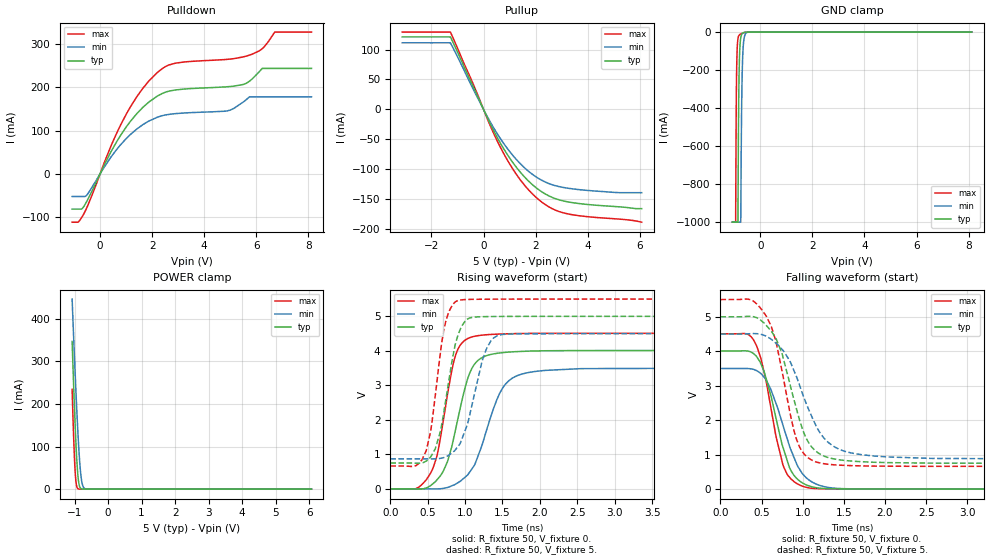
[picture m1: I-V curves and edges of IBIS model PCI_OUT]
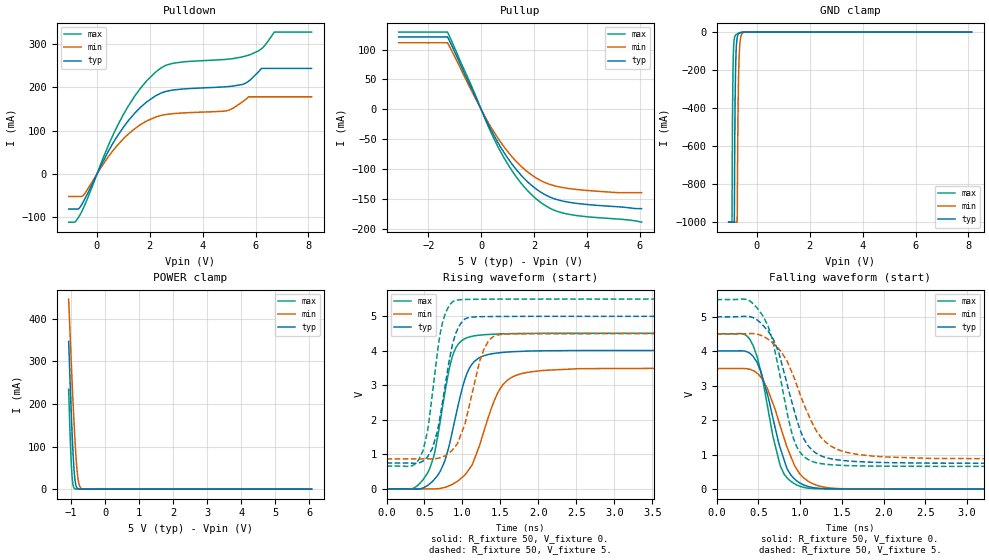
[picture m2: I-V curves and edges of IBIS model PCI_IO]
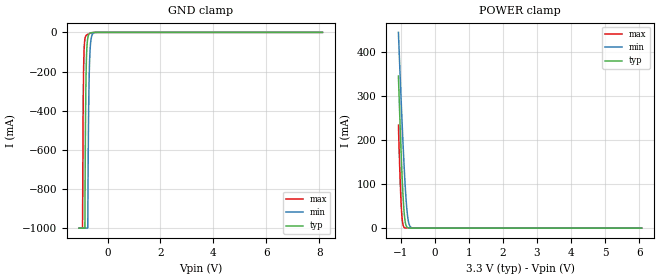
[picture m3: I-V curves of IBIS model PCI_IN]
|   IBIS Model for Tsi382 PBGA Package
[IBIS Ver]   3.2
[Disclaimer] This model is subject to change.
   Integrated Device Technology, Inc. ("IDT") hereby grants the
   user of this IBIS model a non-exclusive, nontransferable
   license to use this IBIS model under the following terms. The
   user is granted this license only to use the IBIS model and is
   not granted rights to sell, copy (except as needed to run the
   IBIS model), rent, lease or sub-license the IBIS model in
   whole or in part, or in modified form to anyone. The User may
   modify the IBIS model to suit its specific applications, but
   rights to derivative works and such modifications shall belong
   to IDT. This IBIS model is provided on an AS IS" basis and IDT
   makes absolutely no warranty with respect to the information
   contained herein. IDT DISCLAIMS AND CUSTOMER WAIVES ALL
   WARRANTIES, EXPRESS AND IMPLIED, INCLUDING WARRANTIES OF
   MERCHANTABILITY AND FITNESS FOR A PARTICULAR PURPOSE. THE
   ENTIRE RISK AS TO QUALITY AND PERFORMANCE IS WITH THE USER
   ACCORDINGLY, IN NO EVENT SHALL IDT BE LIABLE FOR ANY DIRECT OR
   INDIRECT DAMAGES, WHETHER IN CONTRACT OR TORT, INCLUDING ANY
   LOST PROFITS OR OTHER INCIDENTAL, CONSEQUENTIAL, EXEMPLARY, OR
   PUNITIVE DAMAGES ARISING OUT OF THE USE OR APPLICATION OF THE
   IBIS model. Further, IDT reserves the right to make changes
   without notice to any product herein to improve reliability,
   function, or design. IDT does not convey any license under
   patent rights or any other intellectual property rights,
   including those of third parties. IDT is not obligated to
   provide maintenance or support for the licensed IBIS model.
[Copyright]   Copyright 2009, Integrated Device Technology, Inc. all
   rights reserved.
[File Name]   tsi382_5vpci_pbga.ibs
[File Rev]   1.1
[Source]   Developed by:
   Tundra Semiconductor
   603 March Rd.
   Ottawa ON,  K2K 2M5
   www.tundra.com
[Notes]
   Revision History
   Rev 1.0
   - 02/25/2009 Inital Release. IBIS model generated from
   SPICE model extraction. AP
   Rev 1.1
   - 08/31/2009, Updated with IDT formatting. IT
[Component] Tsi382
[Manufacturer] Integrated Device Technology, Inc.
|   typ   min   max
[Package]
R_pkg   218m   168m   293m
L_pkg   3.31nH   2.38nH   5.22nH
C_pkg   0.61pF   0.39pF   1.00pF
[Pin]  signal_name   model_name   R_pin   L_pin   C_pin
E9   GPIO[0]   NC   236.1m   4.0nh   0.67pf
D8   GPIO[1]   NC   212.2m   2.7nh   0.48pf
C9   GPIO[2]   NC   234.6m   3.5nh   0.63pf
D9   GPIO[3]   NC   216.8m   2.8nh   0.52pf
K4   JTAG_TCK   JTAG_IN   260.7m   4.2nh   0.79pf
M3   JTAG_TDI   JTAG_IN   201.1m   2.9nh   0.49pf
K3   JTAG_TDO   JTAG_OUT   199.0m   2.7nh   0.43pf
M12   JTAG_TMS   JTAG_IN   226.1m   3.3nh   0.58pf
K9   JTAG_TRSTn   JTAG_IN   217.8m   3.2nh   0.61pf
B1   PCI_AD[0]   PCI_IO   230.1m   3.2nh   0.65pf
C2   PCI_AD[1]   PCI_IO   218.5m   3.2nh   0.61pf
E1   PCI_AD[10]   PCI_IO   185.3m   2.6nh   0.48pf
G1   PCI_AD[11]   PCI_IO   180.2m   2.5nh   0.45pf
H3   PCI_AD[12]   PCI_IO   221.4m   3.4nh   0.66pf
H1   PCI_AD[13]   PCI_IO   187.1m   2.6nh   0.47pf
H4   PCI_AD[14]   PCI_IO   247.9m   4.2nh   0.80pf
J1   PCI_AD[15]   PCI_IO   197.3m   2.8nh   0.54pf
J5   PCI_AD[16]   PCI_IO   223.4m   3.4nh   0.56pf
J7   PCI_AD[17]   PCI_IO   203.3m   3.1nh   0.63pf
L6   PCI_AD[18]   PCI_IO   199.4m   2.9nh   0.57pf
M6   PCI_AD[19]   PCI_IO   177.7m   2.5nh   0.45pf
F4   PCI_AD[2]   PCI_IO   288.0m   5.2nh   1.00pf
K6   PCI_AD[20]   PCI_IO   217.9m   3.4nh   0.66pf
K7   PCI_AD[21]   PCI_IO   221.0m   3.6nh   0.67pf
M8   PCI_AD[22]   PCI_IO   188.5m   2.8nh   0.50pf
K8   PCI_AD[23]   PCI_IO   231.0m   3.7nh   0.72pf
M10   PCI_AD[24]   PCI_IO   215.9m   3.0nh   0.62pf
L10   PCI_AD[25]   PCI_IO   215.6m   3.1nh   0.65pf
L8   PCI_AD[26]   PCI_IO   168.3m   2.3nh   0.42pf
M11   PCI_AD[27]   PCI_IO   215.8m   3.0nh   0.62pf
H9   PCI_AD[28]   PCI_IO   286.5m   4.9nh   0.98pf
K12   PCI_AD[29]   PCI_IO   202.0m   3.0nh   0.55pf
E3   PCI_AD[3]   PCI_IO   281.6m   4.6nh   0.97pf
J12   PCI_AD[30]   PCI_IO   188.9m   2.7nh   0.50pf
L12   PCI_AD[31]   PCI_IO   222.0m   3.0nh   0.63pf
E2   PCI_AD[4]   PCI_IO   213.7m   3.4nh   0.63pf
F2   PCI_AD[5]   PCI_IO   168.6m   2.4nh   0.43pf
D1   PCI_AD[6]   PCI_IO   200.8m   2.8nh   0.55pf
D3   PCI_AD[7]   PCI_IO   271.0m   4.2nh   0.83pf
F1   PCI_AD[8]   PCI_IO   177.9m   2.5nh   0.44pf
G4   PCI_AD[9]   PCI_IO   236.4m   3.9nh   0.76pf
F3   PCI_CBEn[0]   PCI_IO   222.6m   3.5nh   0.68pf
J3   PCI_CBEn[1]   PCI_IO   243.9m   4.0nh   0.76pf
M4   PCI_CBEn[2]   PCI_IO   190.9m   2.8nh   0.48pf
L9   PCI_CBEn[3]   PCI_IO   227.1m   3.3nh   0.70pf
B12   PCI_CLK   PCI_IN   218.9m   3.1nh   0.59pf
H10   PCI_CLKO[0]   PCI_OUT   246.1m   4.2nh   0.80pf
B2   PCI_CLKO[1]   PCI_OUT   240.6m   3.3nh   0.65pf
J9   PCI_CLKO[2]   PCI_OUT   230.0m   3.2nh   0.57pf
J8   PCI_CLKO[3]   PCI_OUT   276.0m   4.4nh   0.83pf
A12   PCI_CLKO[4]   PCI_OUT   229.3m   3.3nh   0.62pf
M2   PCI_DEVSELn   PCI_IO   225.9m   3.1nh   0.60pf
M5   PCI_FRAMEn   PCI_IO   182.0m   2.6nh   0.46pf
G9   PCI_GNTn[0]   PCI_IO   235.6m   4.0nh   0.76pf
F12   PCI_GNTn[1]   PCI_OUT   178.7m   2.6nh   0.46pf
F11   PCI_GNTn[2]   PCI_OUT   206.3m   3.1nh   0.60pf
E10   PCI_GNTn[3]   PCI_OUT   252.2m   4.1nh   0.82pf
D12   PCI_INTAn   PCI_IN   195.5m   2.7nh   0.54pf
F9   PCI_INTBn   PCI_IN   253.9m   4.4nh   0.84pf
C10   PCI_INTCn   PCI_IN   242.6m   3.9nh   0.75pf
C12   PCI_INTDn   PCI_IN   217.7m   3.2nh   0.59pf
L5   PCI_IRDYn   PCI_IO   205.3m   3.0nh   0.58pf
L3   PCI_LOCKn   PCI_OUT   194.1m   2.7nh   0.48pf
B11   PCI_M66EN   PCI_IN   244.4m   3.5nh   0.71pf
K1   PCI_PAR   PCI_IO   210.2m   2.9nh   0.52pf
J4   PCI_PERRn   PCI_IO   272.8m   4.5nh   0.84pf
H12   PCI_PMEn   PCI_IN   180.5m   2.5nh   0.45pf
F10   PCI_REQn[0]   PCI_IO   204.0m   3.2nh   0.62pf
J10   PCI_REQn[1]   PCI_IN   266.6m   4.2nh   0.82pf
G10   PCI_REQn[2]   PCI_IN   183.1m   2.7nh   0.52pf
H11   PCI_REQn[3]   PCI_IN   204.4m   2.9nh   0.58pf
E12   PCI_RSTn   PCI_OUT   184.7m   2.7nh   0.47pf
J2   PCI_SERRn   PCI_IO   187.1m   2.5nh   0.48pf
J6   PCI_STOPn   PCI_IO   275.1m   5.0nh   0.92pf
K5   PCI_TRDYn   PCI_IO   190.6m   2.7nh   0.53pf
B9   PCIE_PERSTn   NC   254.1m   4.2nh   0.70pf
A8   PCIE_REFCLK_n   NC   188.2m   2.9nh   0.40pf
B8   PCIE_REFCLK_p   NC   188.9m   2.8nh   0.39pf
A11   PCIE_REXT   NC   227.9m   3.5nh   0.75pf
B6   PCIE_RXD_n   NC   190.9m   2.7nh   0.45pf
A6   PCIE_RXD_p   NC   192.5m   2.7nh   0.41pf
B4   PCIE_TXD_n   NC   189.6m   2.9nh   0.41pf
A4   PCIE_TXD_p   NC   186.6m   2.8nh   0.39pf
K11   PWRUP_EN_ARB   GEN33_IN   261.2m   3.8nh   0.82pf
L1   PWRUP_PLL_BYPASS   GEN33_IN   240.0m   3.4nh   0.62pf
A2   SR_CLK   NC   242.9m   3.3nh   0.61pf
D4   SR_CSn   NC   216.3m   2.8nh   0.57pf
A3   SR_DIN   NC   209.3m   2.8nh   0.45pf
E4   SR_DOUT   NC   293.9m   4.8nh   0.88pf
D7   TEST_BCE   NC   225.6m   2.8nh   0.51pf
C3   TEST_BIDR_CTL   NC   216.2m   2.9nh   0.53pf
B3   TEST_ON   NC   223.2m   3.2nh   0.53pf
E5   VDD   POWER
E8   VDD   POWER
F6   VDD   POWER
F7   VDD   POWER
G6   VDD   POWER
G7   VDD   POWER
H5   VDD   POWER
H8   VDD   POWER
D2   VDD_PCI   POWER
D11   VDD_PCI   POWER
E11   VDD_PCI   POWER
G2   VDD_PCI   POWER
G11   VDD_PCI   POWER
H2   VDD_PCI   POWER
J11   VDD_PCI   POWER
K2   VDD_PCI   POWER
L4   VDD_PCI   POWER
L7   VDD_PCI   POWER
L11   VDD_PCI   POWER
B5   VDD_PCIE   POWER
B7   VDD_PCIE   POWER
C4   VDD_PCIE   POWER
C8   VDD_PCIE   POWER
C6   VDDA_PCIE   POWER
D6   VDDA_PCIE   POWER
B10   VDDA_PLL   POWER
C11   VIO_PCI   POWER
L2   VIO_PCI   POWER
M9   VIO_PCI   POWER
A1   VSS   GND
A5   VSS   GND
A7   VSS   GND
A9   VSS   GND
C1   VSS   GND
C5   VSS   GND
C7   VSS   GND
D5   VSS   GND
D10   VSS   GND
E6   VSS   GND
E7   VSS   GND
F5   VSS   GND
F8   VSS   GND
G3   VSS   GND
G5   VSS   GND
G8   VSS   GND
G12   VSS   GND
H6   VSS   GND
H7   VSS   GND
K10   VSS   GND
M1   VSS   GND
M7   VSS   GND
A10   VSSA_PLL   GND
| Models and submodels in the file (6): PCI_OUT (Output), PCI_IO (I/O), PCI_IN (Input), JTAG_IN (Input), JTAG_OUT (Output), GEN33_IN (Input)
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[Model]   PCI_OUT
Model_type  Output
C_comp 4.536p 4.202p 4.874p
Polarity   Non-Inverting
Enable   Active-High
Vmeas =   1.32V
Cref =   10pF
Rref =   50
Vref=   0.0V
[Temperature Range]   27.0   125.0   -40.0
[Voltage Range] 5. 4.5 5.5
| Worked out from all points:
|   slope of the pulldown table from 0 to 0.75 V, typ, clamps not added: 8.81 ohm
|   slope of the pullup table from 0 to 0.75 V, typ, clamps not added: 11.8 ohm
|   GND clamp passes 1 mA (typ) near -0.58 V on its own axis
|   POWER clamp passes 1 mA (typ) near -0.80 V on its own axis
|   rising waveform, R_fixture 50, V_fixture 0.: 20-80 % time 271ps typ, 341ps min, 223ps max; typ from 0 V to 4.01 V
|   rising waveform, R_fixture 50, V_fixture 5.: 20-80 % time 204ps typ, 254ps min, 174ps max; typ from 0.748 V to 5 V
|   falling waveform, R_fixture 50, V_fixture 0.: 20-80 % time 260ps typ, 305ps min, 229ps max; typ from 4.01 V to 0 V
|   falling waveform, R_fixture 50, V_fixture 5.: 20-80 % time 307ps typ, 393ps min, 259ps max; typ from 5 V to 0.748 V
[Pulldown]
-1.072V   -80.93mA   -51.78mA   -111mA
-830.1mV  -80.93mA   -51.78mA   -110.2mA
-625.6mV  -75.05mA   -51.78mA   -92.1mA
425mV     51.67mA    39.35mA    65.16mA
1.011V    108.6mA    81.72mA    138.1mA
2.21V     179.7mA    130.8mA    234.1mA
2.879V    193.3mA    138.9mA    254.9mA
4.887V    200.8mA    145.2mA    263.9mA
5.761V    214.7mA    177.7mA    274.1mA
6.226V    243mA      177.7mA    288.2mA
6.71V     243mA      177.7mA    326.7mA
8.123V    243mA      177.7mA    326.7mA
[Pullup]
-3.123V   121mA      111.2mA    129.1mA
-1.273V   121mA      111.2mA    129.1mA
-408.1mV  39.21mA    34.71mA    43.33mA
103.2mV   -9.96mA    -8.61mA    -11.21mA
754mV     -64.09mA   -55.48mA   -71.94mA
1.433V    -105.7mA   -91.4mA    -118.6mA
1.786V    -121.9mA   -105.2mA   -136.8mA
2.186V    -135.9mA   -116.9mA   -152.8mA
2.725V    -148.2mA   -126.7mA   -167.3mA
3.264V    -154.4mA   -131.5mA   -174.5mA
4.984V    -161.7mA   -138.3mA   -182.2mA
6.072V    -165.4mA   -138.8mA   -188mA
[GND Clamp]
-1.072V   -1A        -1A        -1A
-946.2mV  -1A        -1A        -1A
-927.6mV  -1A        -1A        -477.7mA
-913.6mV  -1A        -1A        -259.6mA
-857.8mV  -1A        -1A        -35.04mA
-829.9mV  -387.1mA   -1A        -20.17mA
-792.7mV  -109.1mA   -1A        -13.52mA
-750.8mV  -31.16mA   -1A        -10.02mA
-718.2mV  -13.49mA   -425.6mA   -7.927mA
-681mV    -5.936mA   -150.7mA   -5.835mA
-541.4mV  -487.9uA   -4.567mA   -875.4uA
8.123V    0A         0A         0A
[Power Clamp]
-1.072V   346.3mA    445.7mA    234.2mA
-1.025V   239mA      352.7mA    117.5mA
-985.9mV  158.9mA    279.6mA    47.19mA
-953.7mV  100.9mA    221.8mA    15.32mA
-930mV    65.56mA    181.6mA    5.554mA
-906.4mV  38.32mA    144mA      1.868mA
-865.6mV  11.54mA    86.96mA    261.8uA
-839.8mV  4.741mA    57.78mA    114.1uA
-809.7mV  1.564mA    32.24mA    114.1uA
-764.6mV  288.3uA    10.74mA    114.1uA
-708.7mV  34.28uA    2.193mA    114.1uA
6.072V    0A         0A         0A
[Ramp]
dV/dt_r 2.406/269.779p 2.1/340.819p 2.705/222.777p
dV/dt_f 2.551/306.834p 2.179/393.351p 2.904/258.7p
[Rising Waveform]
R_fixture = 50
V_fixture = 0.
0s        0V         0V         0V
340ps     -4.676mV   86.06uV    4.549mV
540ps     94.69mV    -2.304mV   456.9mV
640ps     301mV      -2.262mV   1.113V
770ps     822.3mV    41.22mV    2.797V
860ps     1.592V     120.4mV    3.781V
1.06ns    3.349V     481.1mV    4.379V
1.46ns    3.937V     2.758V     4.487V
1.71ns    3.979V     3.291V     4.5V
4.91ns    4.01V      3.5V       4.508V
[Rising Waveform]
R_fixture = 50
V_fixture = 5.
V_fixture_min = 4.5
V_fixture_max = 5.5
0s        748.2mV    868.5mV    660.9mV
340ps     743.4mV    868.5mV    668.5mV
480ps     805.4mV    867.5mV    1.103V
610ps     1.216V     870.6mV    2.858V
720ps     2.281V     911.3mV    4.647V
890ps     4.347V     1.186V     5.445V
1.03ns    4.918V     1.86V      5.488V
1.28ns    4.991V     4.027V     5.496V
1.43ns    4.995V     4.436V     5.498V
4.91ns    5V         4.5V       5.5V
[Falling Waveform]
R_fixture = 50
V_fixture = 0.
0s        4.01V      3.5V       4.508V
400ps     3.94V      3.477V     4.342V
530ps     3.418V     3.25V      3.403V
670ps     2.118V     2.522V     1.6V
760ps     1.216V     1.855V     703.3mV
860ps     527.8mV    1.121V     291.2mV
990ps     192.2mV    470.5mV    92.32mV
1.17ns    40.8mV     141mV      16.71mV
1.44ns    9.292mV    19.45mV    6.614mV
4.91ns    8.688uV    23.08uV    4.321uV
[Falling Waveform]
R_fixture = 50
V_fixture = 5.
V_fixture_min = 4.5
V_fixture_max = 5.5
0s        5V         4.5V       5.5V
370ps     5.012V     4.511V     5.491V
560ps     4.742V     4.432V     5.006V
670ps     4.387V     4.245V     4.331V
740ps     3.99V      4.079V     3.529V
920ps     2.368V     3.287V     1.483V
1.14ns    1.146V     1.95V      809.5mV
1.37ns    882.2mV    1.249V     708.4mV
1.71ns    797.4mV    1.002V     675.1mV
4.91ns    748.3mV    869.1mV    660.9mV
[Model]   PCI_IO
Model_type  I/O
C_comp 4.536p 4.202p 4.874p
Polarity   Non-Inverting
Enable   Active-High
Vinl =   0.80V
Vinh =   2.00V
Vmeas =   1.32V
Cref =   10pF
Rref =   150
Vref=   0.0V
[Temperature Range]   27.0   125.0   -40.0
[Voltage Range] 5. 4.5 5.5
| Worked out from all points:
|   slope of the pulldown table from 0 to 0.75 V, typ, clamps not added: 8.81 ohm
|   slope of the pullup table from 0 to 0.75 V, typ, clamps not added: 11.8 ohm
|   GND clamp passes 1 mA (typ) near -0.58 V on its own axis
|   POWER clamp passes 1 mA (typ) near -0.80 V on its own axis
|   rising waveform, R_fixture 50, V_fixture 0.: 20-80 % time 271ps typ, 341ps min, 223ps max; typ from 0 V to 4.01 V
|   rising waveform, R_fixture 50, V_fixture 5.: 20-80 % time 204ps typ, 254ps min, 174ps max; typ from 0.748 V to 5 V
|   falling waveform, R_fixture 50, V_fixture 0.: 20-80 % time 260ps typ, 305ps min, 229ps max; typ from 4.01 V to 0 V
|   falling waveform, R_fixture 50, V_fixture 5.: 20-80 % time 307ps typ, 393ps min, 259ps max; typ from 5 V to 0.748 V
[Pulldown]
-1.072V   -80.93mA   -51.78mA   -111mA
-830.1mV  -80.93mA   -51.78mA   -110.2mA
-625.6mV  -75.05mA   -51.78mA   -92.1mA
425mV     51.67mA    39.35mA    65.16mA
1.011V    108.6mA    81.72mA    138.1mA
2.21V     179.7mA    130.8mA    234.1mA
2.879V    193.3mA    138.9mA    254.9mA
4.887V    200.8mA    145.2mA    263.9mA
5.761V    214.7mA    177.7mA    274.1mA
6.226V    243mA      177.7mA    288.2mA
6.71V     243mA      177.7mA    326.7mA
8.123V    243mA      177.7mA    326.7mA
[Pullup]
-3.123V   121mA      111.2mA    129.1mA
-1.273V   121mA      111.2mA    129.1mA
-408.1mV  39.21mA    34.71mA    43.33mA
103.2mV   -9.96mA    -8.61mA    -11.21mA
754mV     -64.09mA   -55.48mA   -71.94mA
1.433V    -105.7mA   -91.4mA    -118.6mA
1.786V    -121.9mA   -105.2mA   -136.8mA
2.186V    -135.9mA   -116.9mA   -152.8mA
2.725V    -148.2mA   -126.7mA   -167.3mA
3.264V    -154.4mA   -131.5mA   -174.5mA
4.984V    -161.7mA   -138.3mA   -182.2mA
6.072V    -165.4mA   -138.8mA   -188mA
[GND Clamp]
-1.072V   -1A        -1A        -1A
-946.2mV  -1A        -1A        -1A
-927.6mV  -1A        -1A        -477.7mA
-913.6mV  -1A        -1A        -259.6mA
-857.8mV  -1A        -1A        -35.04mA
-829.9mV  -387.1mA   -1A        -20.17mA
-792.7mV  -109.1mA   -1A        -13.52mA
-750.8mV  -31.16mA   -1A        -10.02mA
-718.2mV  -13.49mA   -425.6mA   -7.927mA
-681mV    -5.936mA   -150.7mA   -5.835mA
-541.4mV  -487.9uA   -4.567mA   -875.4uA
8.123V    0A         0A         0A
[Power Clamp]
-1.072V   346.3mA    445.7mA    234.2mA
-1.025V   239mA      352.7mA    117.5mA
-985.9mV  158.9mA    279.6mA    47.19mA
-953.7mV  100.9mA    221.8mA    15.32mA
-930mV    65.56mA    181.6mA    5.554mA
-906.4mV  38.32mA    144mA      1.868mA
-865.6mV  11.54mA    86.96mA    261.8uA
-839.8mV  4.741mA    57.78mA    114.1uA
-809.7mV  1.564mA    32.24mA    114.1uA
-764.6mV  288.3uA    10.74mA    114.1uA
-708.7mV  34.28uA    2.193mA    114.1uA
6.072V    0A         0A         0A
[Ramp]
dV/dt_r 2.406/269.779p 2.1/340.819p 2.705/222.777p
dV/dt_f 2.551/306.834p 2.179/393.351p 2.904/258.7p
[Rising Waveform]
R_fixture = 50
V_fixture = 0.
0s        0V         0V         0V
340ps     -4.676mV   86.06uV    4.549mV
540ps     94.69mV    -2.304mV   456.9mV
640ps     301mV      -2.262mV   1.113V
770ps     822.3mV    41.22mV    2.797V
860ps     1.592V     120.4mV    3.781V
1.06ns    3.349V     481.1mV    4.379V
1.46ns    3.937V     2.758V     4.487V
1.71ns    3.979V     3.291V     4.5V
4.91ns    4.01V      3.5V       4.508V
[Rising Waveform]
R_fixture = 50
V_fixture = 5.
V_fixture_min = 4.5
V_fixture_max = 5.5
0s        748.2mV    868.5mV    660.9mV
340ps     743.4mV    868.5mV    668.5mV
480ps     805.4mV    867.5mV    1.103V
610ps     1.216V     870.6mV    2.858V
720ps     2.281V     911.3mV    4.647V
890ps     4.347V     1.186V     5.445V
1.03ns    4.918V     1.86V      5.488V
1.28ns    4.991V     4.027V     5.496V
1.43ns    4.995V     4.436V     5.498V
4.91ns    5V         4.5V       5.5V
[Falling Waveform]
R_fixture = 50
V_fixture = 0.
0s        4.01V      3.5V       4.508V
400ps     3.94V      3.477V     4.342V
530ps     3.418V     3.25V      3.403V
670ps     2.118V     2.522V     1.6V
760ps     1.216V     1.855V     703.3mV
860ps     527.8mV    1.121V     291.2mV
990ps     192.2mV    470.5mV    92.32mV
1.17ns    40.8mV     141mV      16.71mV
1.44ns    9.292mV    19.45mV    6.614mV
4.91ns    8.688uV    23.08uV    4.321uV
[Falling Waveform]
R_fixture = 50
V_fixture = 5.
V_fixture_min = 4.5
V_fixture_max = 5.5
0s        5V         4.5V       5.5V
370ps     5.012V     4.511V     5.491V
560ps     4.742V     4.432V     5.006V
670ps     4.387V     4.245V     4.331V
740ps     3.99V      4.079V     3.529V
920ps     2.368V     3.287V     1.483V
1.14ns    1.146V     1.95V      809.5mV
1.37ns    882.2mV    1.249V     708.4mV
1.71ns    797.4mV    1.002V     675.1mV
4.91ns    748.3mV    869.1mV    660.9mV
|   MODEL PCI_IN
[Model]   PCI_IN
Model_type  Input
C_comp 4.536p 4.202p 4.874p
Polarity   Non-Inverting
Enable   Active-High
Vinl =   0.80V
Vinh =   2.00V
[Temperature Range]   27.0   125.0   -40.0
[POWER Clamp Reference]   3.30V   3.00V   3.60V
[GND Clamp Reference]   0.00V   0.00V   0.00V
[Voltage Range] 3.3 3. 3.6
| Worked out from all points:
|   GND clamp passes 1 mA (typ) near -0.58 V on its own axis
|   POWER clamp passes 1 mA (typ) near -0.80 V on its own axis
[GND Clamp]
-1.072V   -1A        -1A        -1A
-946.2mV  -1A        -1A        -1A
-927.6mV  -1A        -1A        -477.7mA
-913.6mV  -1A        -1A        -259.6mA
-857.8mV  -1A        -1A        -35.04mA
-829.9mV  -387.1mA   -1A        -20.17mA
-792.7mV  -109.1mA   -1A        -13.52mA
-750.8mV  -31.16mA   -1A        -10.02mA
-718.2mV  -13.49mA   -425.6mA   -7.927mA
-681mV    -5.936mA   -150.7mA   -5.835mA
-541.4mV  -487.9uA   -4.567mA   -875.4uA
8.123V    0A         0A         0A
[Power Clamp]
-1.072V   346.3mA    445.7mA    234.2mA
-1.025V   239mA      352.7mA    117.5mA
-985.9mV  158.9mA    279.6mA    47.19mA
-953.7mV  100.9mA    221.8mA    15.32mA
-930mV    65.56mA    181.6mA    5.554mA
-906.4mV  38.32mA    144mA      1.868mA
-865.6mV  11.54mA    86.96mA    261.8uA
-839.8mV  4.741mA    57.78mA    114.1uA
-809.7mV  1.564mA    32.24mA    114.1uA
-764.6mV  288.3uA    10.74mA    114.1uA
-708.7mV  34.28uA    2.193mA    114.1uA
6.072V    0A         0A         0A
